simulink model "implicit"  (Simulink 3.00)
settings: Solver=ode5  StartTime=0.0  StopTime=10  FixedStep=0.05  MaxStep=0.05  RelTol=1e-3  AbsTol=1e-3
libraries: simulink3 x1

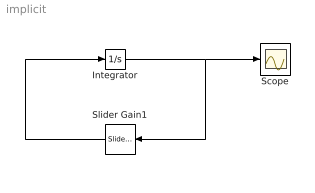
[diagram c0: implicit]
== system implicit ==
  Integrator : Integrator  ExternalReset=none  InitialConditionSource=internal  InitialCondition=1  LimitOutput=off  UpperSaturationLimit=inf  LowerSaturationLimit=-inf  ShowSaturationPort=off  ShowStatePort=off  AbsoluteTolerance=auto
  Scope : Scope
  Slider Gain1 : simulink3/Math/Slider Gain  Orientation=left  low=-1  gain=-0.305  high=0
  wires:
  Integrator/1 -> Slider Gain1/1, Scope/1
  Slider Gain1/1 -> Integrator/1
